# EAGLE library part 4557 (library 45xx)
1 to 64 bit variable length SHIFT REGISTER
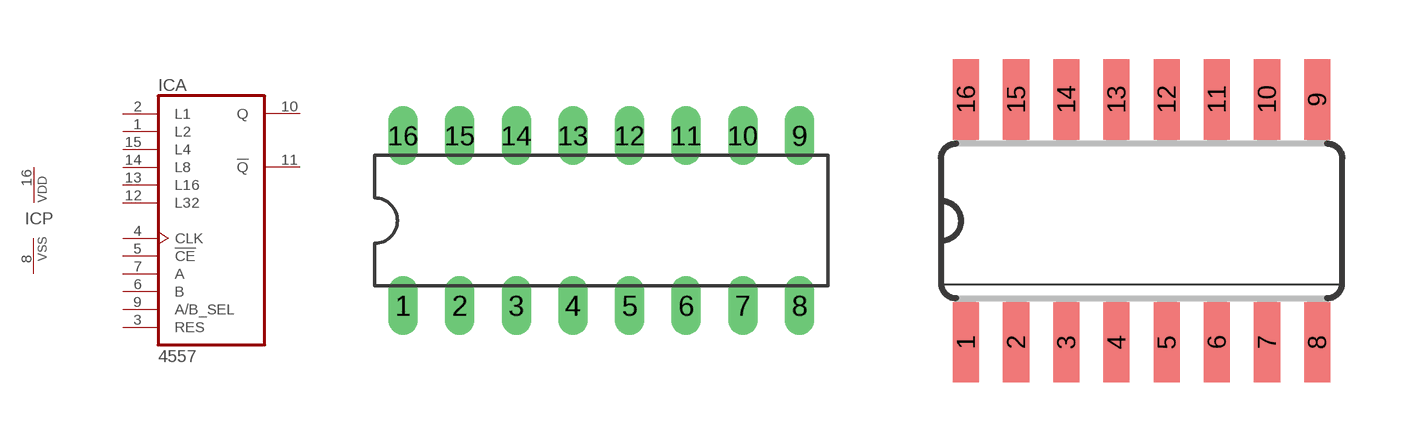
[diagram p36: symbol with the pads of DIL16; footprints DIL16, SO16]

Designator prefix IC; gates A=4557 P=PWRN

## 4557N  [DIL16]
1  A:L2  in
2  A:L1  in
3  A:RES  in
4  A:CLK  in
5  A:!CE  in
6  A:B  in
7  A:A  in
8  P:VSS  pwr
9  A:A/B_SEL  in
10  A:Q  out
11  A:!Q  out
12  A:L32  in
13  A:L16  in
14  A:L8  in
15  A:L4  in
16  P:VDD  pwr

## 4557D  [SO16]
Pads as for DIL16

## Footprint DIL16 (pad centres in mm)
Dual In Line Package
drill 0.813 long: 1 -8.89,-3.81; 2 -6.35,-3.81; 3 -3.81,-3.81; 4 -1.27,-3.81; 5 1.27,-3.81; 6 3.81,-3.81; 7 6.35,-3.81; 8 8.89,-3.81; 9 8.89,3.81; 10 6.35,3.81; 11 3.81,3.81; 12 1.27,3.81; 13 -1.27,3.81; 14 -3.81,3.81; 15 -6.35,3.81; 16 -8.89,3.81

## Footprint SO16 (pad centres in mm)
Small Outline package 150 mil
smd 0.66 x 2.032: 1 -4.445,-3.073; 2 -3.175,-3.073; 3 -1.905,-3.073; 4 -0.635,-3.073; 5 0.635,-3.073; 6 1.905,-3.073; 7 3.175,-3.073; 8 4.445,-3.073; 9 4.445,3.073; 10 3.175,3.073; 11 1.905,3.073; 12 0.635,3.073; 13 -0.635,3.073; 14 -1.905,3.073; 15 -3.175,3.073; 16 -4.445,3.073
